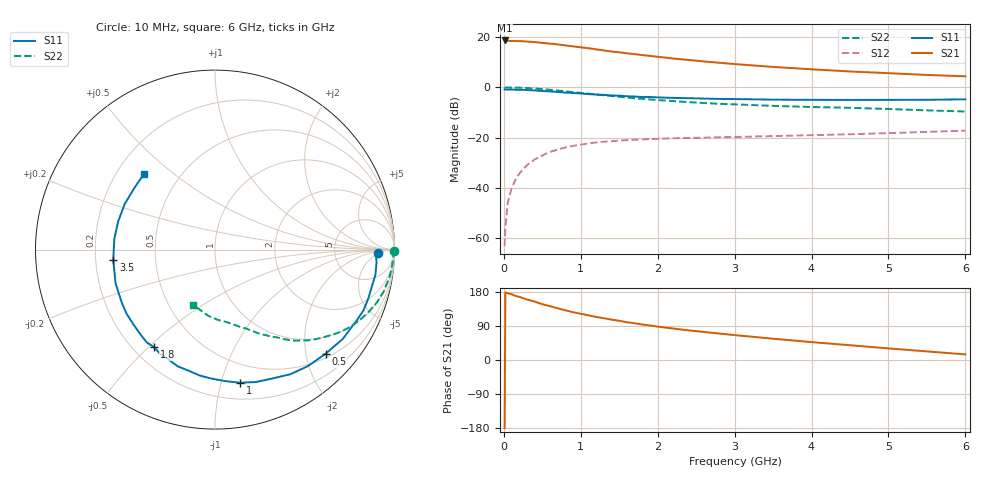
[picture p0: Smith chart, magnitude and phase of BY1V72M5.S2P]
! SIEMENS Small Signal Semiconductors
! BFY420
! Si NPN RF SIEGET Grounded Emitter Transistor in MICRO-X
! VCE = 1.75 V  IC = 2.5 mA
! Common Emitter S-Parameters:  October  1996
# GHz  S  MA  R  50
!  f  S11  S21  S12  S22
! GHz  MAG  ANG  MAG  ANG  MAG  ANG  MAG  ANG
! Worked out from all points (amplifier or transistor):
!   36 points, 10 MHz to 6 GHz, reference 50 ohm
!   highest |S21| = 18.6 dB at 10 MHz (marker M1)
!   |S21| within 3 dB of that: start of sweep to 1.074 GHz
!   unconditionally stable (mu >= 1): 3.804 GHz to end of sweep
!   at 250 MHz: K = 0.06, MSG = 25.4 dB, |S12| = -32.5 dB
!   at 1.4 GHz: K = 0.34, MSG = 17.8 dB, |S12| = -21.4 dB
!   at 6 GHz: K = 1.22, MAG = 7.9 dB, |S12| = -17.2 dB
!   S11 on the Smith chart (normalised r, x): 10 MHz: 20, -4; 500 MHz: 0.59, -2.40; 1 GHz: 0.33, -1.15; 1.8 GHz: 0.28, -0.52; 3.5 GHz: 0.27, -0.05; 6 GHz: 0.31, +0.40
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0.01  0.91 -1.2  8.528 -179.7  0.0007 95.3  0.9951 -0.5
0.02  0.8973 -1.8  8.455 178.3  0.0017 98.8  0.9877 -0.9
0.05  0.9031 -4.7  8.36 176.1  0.005 87.8  0.9945 -2.3
0.1  0.9047 -9.0  8.341 173.6  0.0098 82.8  0.9912 -4.8
0.15  0.8977 -13.4  8.301 169.2  0.0145 81.8  0.9873 -7.1
0.2  0.8964 -17.8  8.276 166.7  0.0192 80.5  0.9835 -9.3
0.25  0.8938 -22.3  8.224 163.1  0.0236 76.9  0.9742 -11.6
0.4  0.8686 -35.0  7.93 154.2  0.0368 69.9  0.9471 -18.4
0.5  0.8463 -43.3  7.621 147.2  0.0444 66.0  0.9213 -22.5
0.7  0.8116 -58.8  7.124 136.5  0.0583 57.6  0.8657 -30.0
0.9  0.7721 -72.9  6.504 126.1  0.0687 50.4  0.8025 -36.4
1  0.7546 -79.4  6.215 121.9  0.0728 47.2  0.7738 -39.3
1.1  0.734 -85.9  5.977 117.8  0.077 44.6  0.7468 -42.1
1.4  0.6895 -102.7  5.136 106.6  0.085 37.6  0.6741 -48.8
1.6  0.6638 -113.2  4.738 99.7  0.0894 33.9  0.6273 -52.6
1.8  0.6407 -122.0  4.368 93.7  0.0921 30.9  0.5898 -55.7
2.2  0.6169 -137.5  3.738 83.1  0.0974 26.2  0.5344 -61.7
2.8  0.5884 -156.1  3.074 69.8  0.102 21.9  0.4699 -68.9
3.5  0.5696 -174.3  2.541 56.2  0.1077 19.1  0.4285 -76.3
4.5  0.5619 163.7  2.065 39.0  0.1169 16.1  0.3915 -87.8
5.5  0.5654 142.8  1.761 22.7  0.1301 13.6  0.3486 -102.9
6  0.5777 133.3  1.653 14.7  0.1381 12.0  0.3308 -111.8
